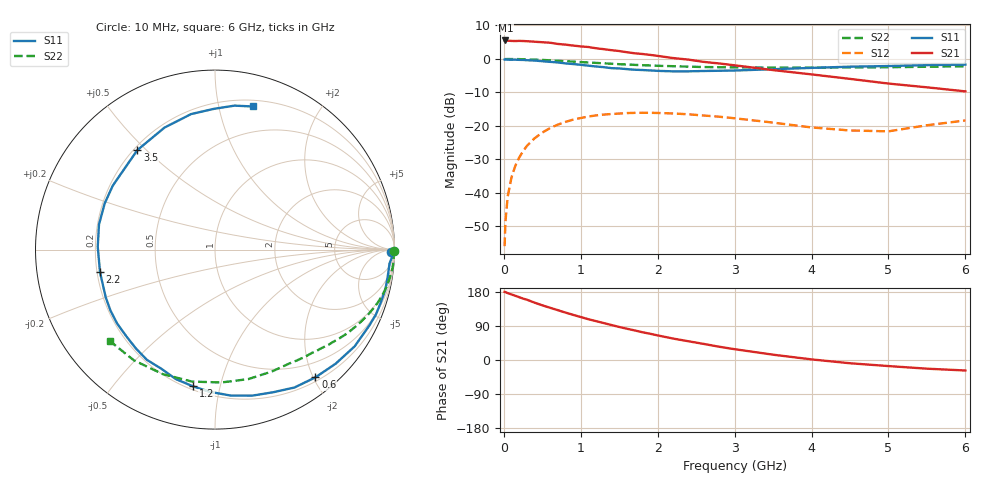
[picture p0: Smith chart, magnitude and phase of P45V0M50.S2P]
! SIEMENS Small Signal Semiconductors
! BFP182
! Si NPN RF Bipolar Junction Transistor in SOT143
! VCE = 5 V  IC = 0.5 mA
! Common Emitter S-Parameters:  March  1996
# GHz  S  MA  R  50
!  f  S11  S21  S12  S22
! GHz  MAG  ANG  MAG  ANG  MAG  ANG  MAG  ANG
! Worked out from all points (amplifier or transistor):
!   36 points, 10 MHz to 6 GHz, reference 50 ohm
!   highest |S21| = 5.5 dB at 20 MHz (marker M1)
!   |S21| within 3 dB of that: start of sweep to 1.436 GHz
!   unconditionally stable (mu >= 1): 2.953 GHz to end of sweep
!   at 250 MHz: K = 0.09, MSG = 16.5 dB, |S12| = -27.6 dB
!   at 1.4 GHz: K = 0.49, MSG = 9.5 dB, |S12| = -16.4 dB
!   at 6 GHz: K = 1.23, MAG = 1.4 dB, |S12| = -18.4 dB
!   S11 on the Smith chart (normalised r, x): 10 MHz: 70, -56; 600 MHz: 0.26, -2.03; 1.2 GHz: 0.22, -0.83; 2.2 GHz: 0.21, -0.09; 3.5 GHz: 0.21, +0.47; 6 GHz: 0.25, +1.26
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0.01  0.9826 -0.8  1.871 179.7  0.0016 83.7  0.9986 -0.3
0.02  0.9904 -1.9  1.889 179.3  0.0036 91.9  0.9947 -0.6
0.05  0.9755 -4.5  1.872 176.5  0.0088 89.6  0.9981 -1.5
0.1  0.9741 -8.7  1.859 173.0  0.0171 83.8  0.9957 -3.1
0.15  0.975 -13.3  1.851 169.4  0.0255 81.1  0.9956 -4.7
0.2  0.9693 -17.9  1.862 165.7  0.0338 78.8  0.994 -6.2
0.3  0.9579 -26.3  1.841 159.1  0.0504 72.4  0.9858 -9.4
0.4  0.9466 -34.7  1.809 151.3  0.0654 67.4  0.9777 -12.3
0.6  0.9054 -51.8  1.748 137.9  0.0927 56.2  0.9541 -18.0
0.8  0.8586 -67.7  1.637 125.2  0.1146 46.6  0.9258 -23.2
1.1  0.7933 -92.0  1.507 107.6  0.138 33.3  0.8848 -30.0
1.2  0.7717 -99.1  1.443 102.5  0.1436 29.1  0.8727 -32.2
1.5  0.722 -121.7  1.313 87.2  0.153 18.5  0.8352 -38.0
1.8  0.6833 -142.9  1.187 73.3  0.1573 9.9  0.8073 -43.0
2.2  0.6529 -168.8  1.032 56.6  0.1534 -0.6  0.7795 -50.1
2.8  0.6663 157.3  0.856 35.0  0.1372 -11.6  0.752 -60.9
3.5  0.7031 128.0  0.682 14.0  0.112 -17.6  0.7451 -75.5
4  0.7357 112.5  0.588 1.6  0.0949 -14.0  0.7411 -87.2
4.5  0.7667 100.0  0.504 -8.6  0.0855 -6.8  0.7465 -99.9
5  0.7838 90.6  0.429 -16.0  0.083 7.9  0.7522 -112.8
5.5  0.8094 82.3  0.377 -22.9  0.1023 14.7  0.7647 -126.2
6  0.8244 75.3  0.328 -27.7  0.1207 16.2  0.7767 -139.1
